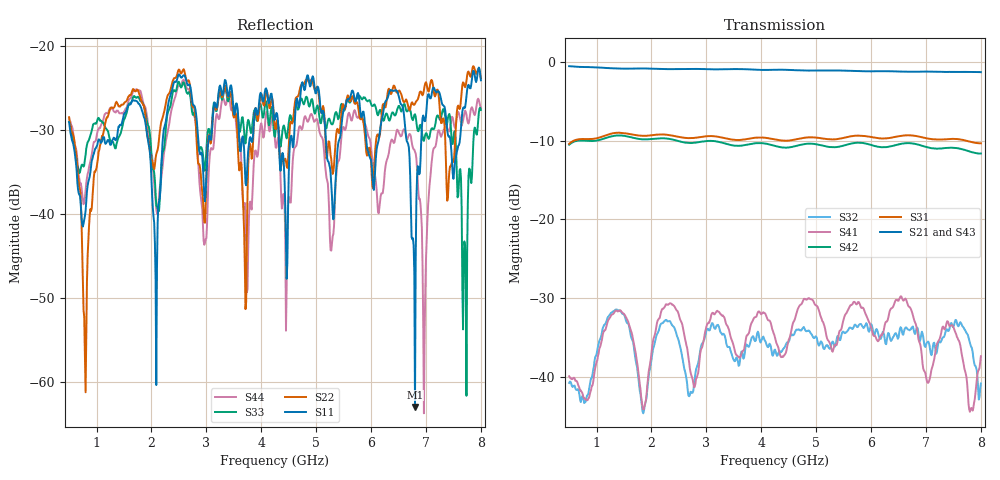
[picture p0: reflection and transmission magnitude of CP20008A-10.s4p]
! Amtery
! Email: info@amtery.com
! Phone: 886-2-2883-7839
! Model Number: CP20008A-10
! 4-port S-parameter measurement data for Bi-Directional Coupler
! Frequency Range: 0.5 GHz to 8 GHz
! Port 1: Input
! Port 2: Output
! Port 3: Coupled Forward
! Port 4: Coupled Reverse
# Hz S ma R 50
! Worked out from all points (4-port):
!   601 points, 500 MHz to 8 GHz, reference 50 ohm
!   strongest paths, dB at 500 MHz, 2.375 GHz, 4.25 GHz, 6.125 GHz, 8 GHz:
!     S21: -0.6, -0.9, -1.0, -1.2, -1.3
!     S43: -0.6, -0.9, -1.0, -1.2, -1.3
!     S31: -10.4, -9.4, -9.9, -9.7, -10.3
!     S42: -10.5, -9.9, -10.7, -10.8, -11.6
!     S41: -39.9, -30.8, -35.0, -35.5, -37.4
!     S32: -40.8, -33.4, -36.5, -34.4, -40.8
!   lowest |S11| = -63.0 dB at 6.8 GHz (marker M1), VSWR 1.00, Z = 49.9 + j0.0245 ohm
!   |S11| at or under -10 dB: start of sweep to end of sweep
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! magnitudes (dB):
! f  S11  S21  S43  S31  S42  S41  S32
! 500 MHz  -29.1  -0.6  -0.6  -10.4  -10.5  -39.9  -40.8
! 787.5 MHz  -40.2  -0.7  -0.7  -9.8  -10.0  -42.7  -43.2
! 1.675 GHz  -26.5  -0.9  -0.9  -9.3  -9.7  -35.6  -36.0
! 6.8 GHz  -63.0  -1.3  -1.3  -9.4  -10.4  -33.1  -34.5
! 6.975 GHz  -28.9  -1.2  -1.2  -9.6  -10.7  -39.3  -36.1
! 7.7 GHz  -27.4  -1.3  -1.3  -10.0  -11.2  -39.0  -33.9
! 8 GHz  -24.1  -1.3  -1.3  -10.3  -11.6  -37.4  -40.8
